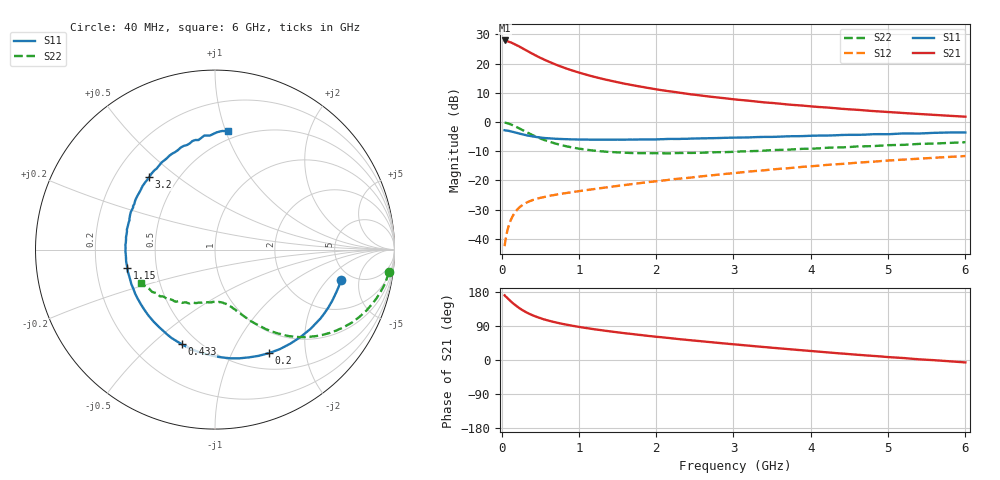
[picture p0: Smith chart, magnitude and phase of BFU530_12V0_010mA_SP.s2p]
! Filename:  P:\Prog\Test\Noise\ATS_data\Testdata_Net\03 Spar\BFU530_APG2013_40_A05_12p0V_010mA_SP_CM01_D.s2p
! Date/Time: Fri 26/Apr/2013 13:03:12
! BFU530_APG2013_40_A05_12p0V_1to25mA_SP_CM01_Bias5_R.s2p
! MDIF S-parameter v. bias file
! BFU530_APG2013_40_A05_12p0V_1to25mA_SP_CM01
! Date/time Wed Apr 24 20:41:12 2013
! VAR V_out= 12.0000
! VAR I_out= 10.0000
! VAR V_in= 0.8048
! VAR I_in= 0.0951
! Device data file deembeded for feedlines and parallel
! Original file: \03 Spar\BFU530_APG2013_40_A05_12p0V_010mA_SP_CM01_R.s2p
! Feed-files: PR047V01_250413_Feed1.s2p, PR047V01_250413_Feed2.s2p
! Parallel-file: PR047V01_250413_Par.s2p
# MHz S MA R 50
!  Freq-MHz  S11-mag  S11-arg  S21-mag  S21-arg  S12-mag  S12-arg  S22-mag  S22-arg
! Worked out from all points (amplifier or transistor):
!   98 points, 40 MHz to 6 GHz, reference 50 ohm
!   highest |S21| = 27.9 dB at 40 MHz (marker M1)
!   |S21| within 3 dB of that: start of sweep to 292.8 MHz
!   unconditionally stable (mu >= 1): 1.835 GHz to 4.109 GHz
!   at 300 MHz: K = 0.30, MSG = 26.4 dB, |S12| = -27.9 dB
!   at 1.6 GHz: K = 0.96, MSG = 17.3 dB, |S12| = -21.5 dB
!   at 6 GHz: K = 0.88, MSG = 6.7 dB, |S12| = -11.6 dB
!   S11 on the Smith chart (normalised r, x): 40 MHz: 4.09, -2.89; 200 MHz: 0.70, -1.41; 433 MHz: 0.41, -0.62; 1.15 GHz: 0.34, -0.09; 3.2 GHz: 0.35, +0.40; 6 GHz: 0.43, +1.02
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40  0.7228 -13.5  24.85 170.7  0.007513 81.1  0.9756 -7.4
50  0.7195 -16.9  24.81 168.1  0.009305 79.9  0.9711 -9.4
120  0.6917 -39.6  23.02 154.8  0.02102 70.6  0.9097 -21.9
160  0.6712 -51.4  21.74 147.9  0.02667 65.7  0.8641 -28.1
200  0.6506 -62.4  20.46 141.5  0.03139 61.6  0.8131 -33.6
240  0.6291 -72.7  19.23 135.6  0.03536 58.0  0.765 -38.4
300  0.6025 -86.1  17.4 128.1  0.04021 53.9  0.6963 -44.4
380  0.5737 -101.2  15.19 120.0  0.04501 49.8  0.6166 -50.7
433  0.5583 -109.5  13.95 115.5  0.04764 48.1  0.5726 -53.9
550  0.5333 -125.2  11.72 107.2  0.05195 45.5  0.4932 -59.6
700  0.5168 -139.7  9.627 99.3  0.05689 44.3  0.4275 -64.6
850  0.508 -151.1  8.133 92.9  0.0613 44.2  0.3815 -68.5
1050  0.5003 -163.4  6.716 85.8  0.06698 44.8  0.3431 -72.8
1150  0.4989 -168.3  6.169 82.7  0.06993 45.3  0.3292 -74.5
1600  0.4989 173.2  4.504 70.5  0.08371 47.0  0.2979 -82.4
2050  0.5072 160.0  3.538 60.4  0.09836 47.9  0.2918 -90.2
2450  0.5206 148.9  2.976 52.0  0.1121 48.0  0.2957 -97.7
3100  0.5423 133.8  2.376 39.6  0.1374 47.1  0.3137 -108.5
3200  0.5455 132.3  2.313 37.8  0.1421 46.8  0.3169 -109.8
4100  0.5856 113.9  1.807 22.1  0.179 42.6  0.3535 -125.5
5200  0.6383 95.3  1.426 5.2  0.2274 35.2  0.4067 -143.4
6000  0.6629 83.7  1.233 -6.4  0.2617 28.5  0.4514 -156.0
